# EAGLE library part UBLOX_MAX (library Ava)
UBLOX MAX
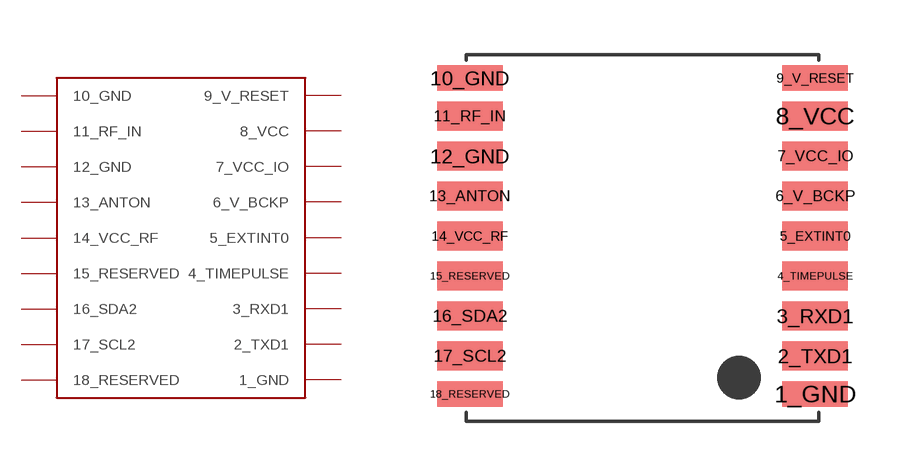
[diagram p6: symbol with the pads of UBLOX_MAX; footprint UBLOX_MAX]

Designator prefix -

## UBLOX_MAX  [UBLOX_MAX]
1_GND  1_GND  pwr
2_TXD1  2_TXD1
3_RXD1  3_RXD1
4_TIMEPULSE  4_TIMEPULSE
5_EXTINT0  5_EXTINT0
6_V_BCKP  6_V_BCKP
7_VCC_IO  7_VCC_IO  pwr
8_VCC  8_VCC  pwr
9_V_RESET  9_V_RESET  pwr
10_GND  10_GND  pwr
11_RF_IN  11_RF_IN
12_GND  12_GND  pwr
13_ANTON  13_ANTON
14_VCC_RF  14_VCC_RF
15_RESERVED  15_RESERVED
16_SDA2  16_SDA2
17_SCL2  17_SCL2
18_RESERVED  18_RESERVED

## Footprint UBLOX_MAX (pad centres in mm)
uBlox MAX
smd 1.8 x 0.7: 1_GND 4.95,-4.4; 9_V_RESET 4.95,4.3; 10_GND -4.55,4.3; 18_RESERVED -4.55,-4.4
smd 1.8 x 0.8: 2_TXD1 4.95,-3.35; 3_RXD1 4.95,-2.25; 4_TIMEPULSE 4.95,-1.15; 5_EXTINT0 4.95,-0.05; 6_V_BCKP 4.95,1.05; 7_VCC_IO 4.95,2.15; 8_VCC 4.95,3.25; 11_RF_IN -4.55,3.25; 12_GND -4.55,2.15; 13_ANTON -4.55,1.05; 14_VCC_RF -4.55,-0.05; 15_RESERVED -4.55,-1.15; 16_SDA2 -4.55,-2.25; 17_SCL2 -4.55,-3.35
